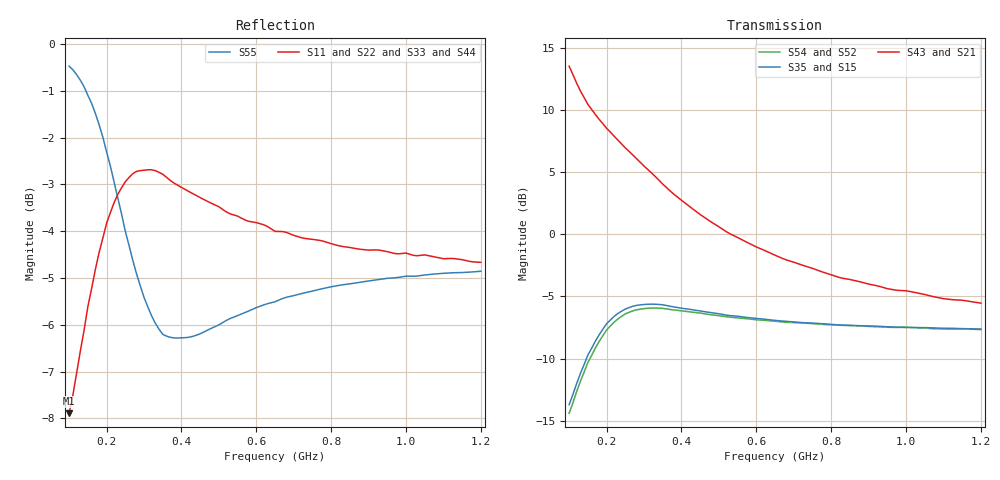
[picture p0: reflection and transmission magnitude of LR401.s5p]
!  POLYFET RF DEVICES
!  LR401
!  Each Side
!  S PARAMETERS
!  VDS=28V, IDQ=600mA
! Date: Wed Apr 07 15:05:08 1999
! SCATTERING PARAMETERS
!AWR Design Environment (2053) Wed Feb 04 15:22:06 2004
!freq-unit  param-type  data-format  keyword  impedance-ohms
# MHz  S  MA  R  50
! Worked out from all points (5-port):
!   111 points, 100 MHz to 1.2 GHz, reference 50 ohm
!   strongest paths, dB at 100 MHz, 370 MHz, 650 MHz, 930 MHz, 1.2 GHz:
!     S43: 13.5, 3.5, -1.7, -4.2, -5.5
!     S21: 13.5, 3.5, -1.7, -4.2, -5.5
!     S35: -13.7, -5.8, -6.9, -7.4, -7.6
!     S15: -13.7, -5.8, -6.9, -7.4, -7.6
!     S54: -14.4, -6.0, -7.0, -7.4, -7.7
!     S52: -14.4, -6.0, -7.0, -7.4, -7.7
!   lowest |S11| = -7.9 dB at 100 MHz (marker M1), VSWR 2.35, Z = 40.4 - j38.4 ohm
!   |S11| at or under -10 dB: nowhere
